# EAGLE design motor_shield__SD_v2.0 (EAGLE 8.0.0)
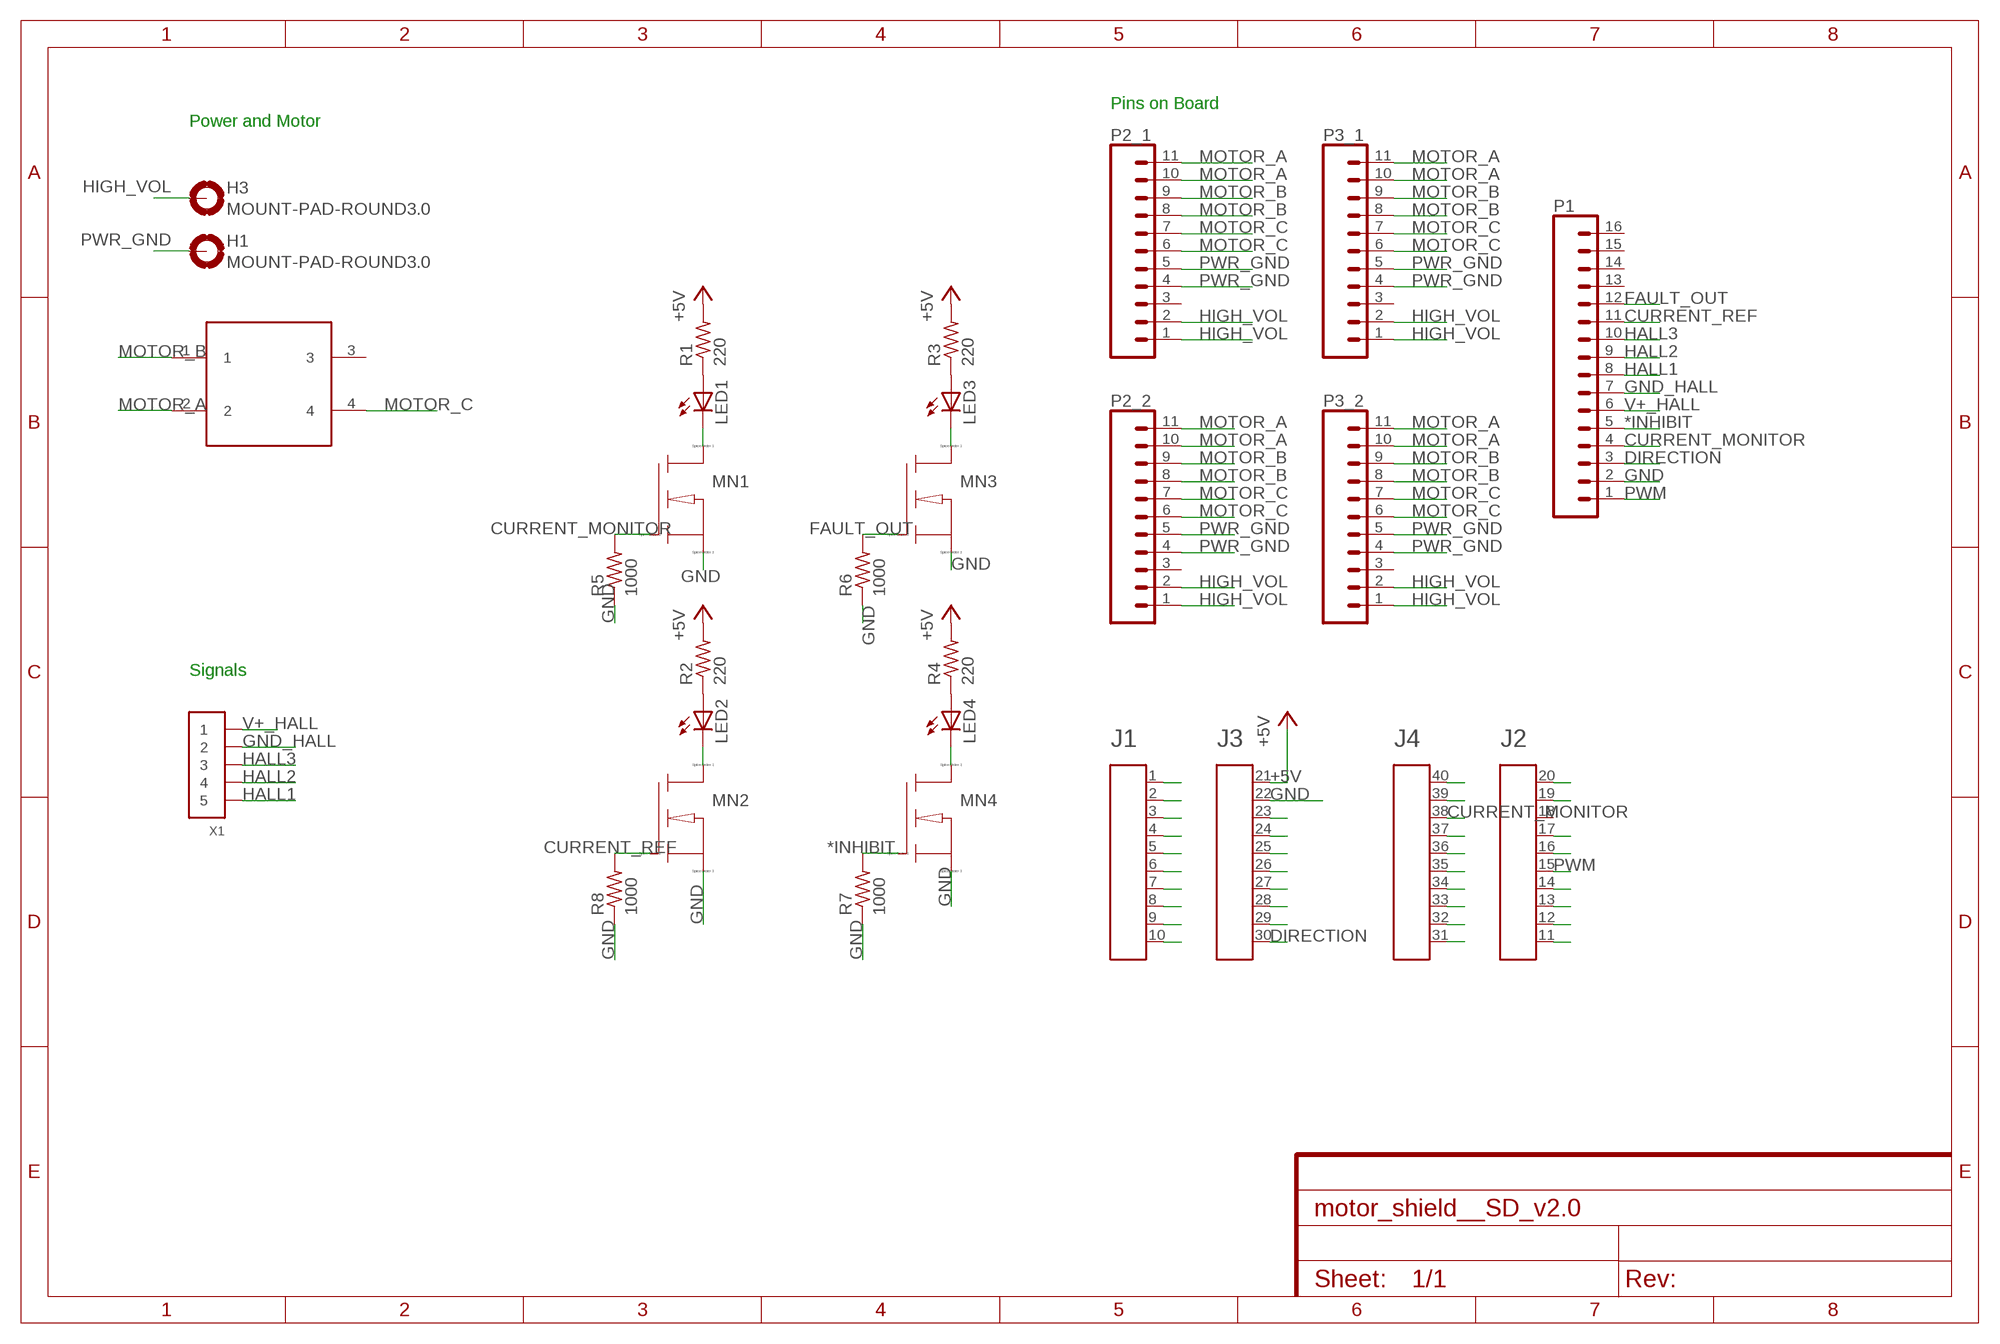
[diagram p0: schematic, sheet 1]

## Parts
A1  HEADER4X10-BOOSTERPACK  [4X10-BOOSTERPACK]
H1  MOUNT-PAD-ROUND3.0  [3,0-PAD]
H3  MOUNT-PAD-ROUND3.0  [3,0-PAD]
LED1  LEDCHIPLED_0805  [CHIPLED_0805]
LED2  LEDCHIPLED_0805  [CHIPLED_0805]
LED3  LEDCHIPLED_0805  [CHIPLED_0805]
LED4  LEDCHIPLED_0805  [CHIPLED_0805]
MN1  NMOS  [SOT23]
MN2  NMOS  [SOT23]
MN3  NMOS  [SOT23]
MN4  NMOS  [SOT23]
P1  CONN_16LOCK  [1X16_LOCK]
P2_1  CONN_11  [1X11]
P2_2  CONN_11  [1X11]
P3_1  CONN_11  [1X11]
P3_2  CONN_11  [1X11]
R1  220  R-US_R0603  [R0603]
R2  220  R-US_R0603  [R0603]
R3  220  R-US_R0603  [R0603]
R4  220  R-US_R0603  [R0603]
R5  1000  R-US_R0603  [R0603]
R6  1000  R-US_R0603  [R0603]
R7  1000  R-US_R0603  [R0603]
R8  1000  R-US_R0603  [R0603]
U$2  MOLEX4CON  [MOLEX4CON]
X1  CONN_5-1-53261  [PB-53261-05]

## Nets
*INHIBIT: MN4.1(G) P1.5 R7.2
+5V: A1.21 R1.2 R2.2 R3.2 R4.2
CURRENT_MONITOR: A1.38 MN1.1(G) P1.4 R5.2
CURRENT_REF: MN2.1(G) P1.11 R8.2
DIRECTION: A1.30 P1.3
FAULT_OUT: MN3.1(G) P1.12 R6.2
GND: A1.22 MN1.2(S) MN2.2(S) MN3.2(S) MN4.2(S) P1.2 R5.1 R6.1 R7.1 R8.1
GND_HALL: P1.7 X1.2
HALL1: P1.8 X1.5
HALL2: P1.9 X1.4
HALL3: P1.10 X1.3
HIGH_VOL: H3.B3,0(MOUNT) P2_1.1 P2_1.2 P2_2.1 P2_2.2 P3_1.1 P3_1.2 P3_2.1 P3_2.2
MOTOR_A: P2_1.10 P2_1.11 P2_2.10 P2_2.11 P3_1.10 P3_1.11 P3_2.10 P3_2.11 U$2.2
MOTOR_B: P2_1.8 P2_1.9 P2_2.8 P2_2.9 P3_1.8 P3_1.9 P3_2.8 P3_2.9 U$2.1
MOTOR_C: P2_1.6 P2_1.7 P2_2.6 P2_2.7 P3_1.6 P3_1.7 P3_2.6 P3_2.7 U$2.4
N$1: LED1.A R1.1
N$2: LED2.A R2.1
N$10: LED3.A R3.1
N$11: LED4.A R4.1
N$15: LED1.C MN1.3(D)
N$16: LED2.C MN2.3(D)
N$30: LED3.C MN3.3(D)
N$41: LED4.C MN4.3(D)
N$46: A1.1
N$47: A1.2
N$48: A1.3
N$49: A1.4
N$50: A1.5
N$51: A1.6
N$52: A1.7
N$53: A1.8
N$54: A1.9
N$55: A1.10
N$58: A1.23
N$59: A1.24
N$60: A1.25
N$61: A1.26
N$62: A1.27
N$63: A1.28
N$64: A1.29
N$66: A1.40
N$67: A1.39
N$69: A1.37
N$70: A1.36
N$71: A1.35
N$72: A1.34
N$73: A1.33
N$74: A1.32
N$75: A1.31
N$76: A1.20
N$77: A1.19
N$79: A1.17
N$80: A1.16
N$82: A1.14
N$83: A1.13
N$84: A1.12
N$85: A1.11
PWM: A1.15 P1.1
PWR_GND: H1.B3,0(MOUNT) P2_1.4 P2_1.5 P2_2.4 P2_2.5 P3_1.4 P3_1.5 P3_2.4 P3_2.5
V+_HALL: P1.6 X1.1
Unconnected: A1.18 P1.13 P1.14 P1.15 P1.16 P2_1.3 P2_2.3 P3_1.3 P3_2.3 U$2.3

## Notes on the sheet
- Pins on Board
- Power and Motor
- Signals

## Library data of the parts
A1 = EAGLE_BoosterPack_Library:HEADER4X10-BOOSTERPACK
H1 H3 = holes:MOUNT-PAD-ROUND: MOUNTING PAD, round
LED1-LED4 = adafruit:LED: LED
MN1-MN4 = sym:NMOS: N-Channel MOSFET transistor
P1 = SparkFun-Connectors:CONN_16: Multi connection point. Often used as Generic Header-pin footprint for 0.1 inch spaced/style header connections On any of the 0.1 inch spaced packages, you can populate with these: Break Away Headers - Straight (PRT-00116) Break Away Male Headers - Right Angle (PRT-00553) Female Headers (PRT-00115)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
P2_1 P2_2 P3_1 P3_2 = SparkFun-Connectors:CONN_11: Multi connection point. Often used as Generic Header-pin footprint for 0.1 inch spaced/style header connections On any of the 0.1 inch spaced packages, you can populate with these: Break Away Headers - Straight (PRT-00116) Break Away Male Headers - Right Angle (PRT-00553) Female Headers (PRT-00115)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
R1-R8 = adafruit:R-US_: RESISTOR, American symbol
U$2 = TREC1:MOLEX4CON
X1 = pel_molex:CONN_5-1

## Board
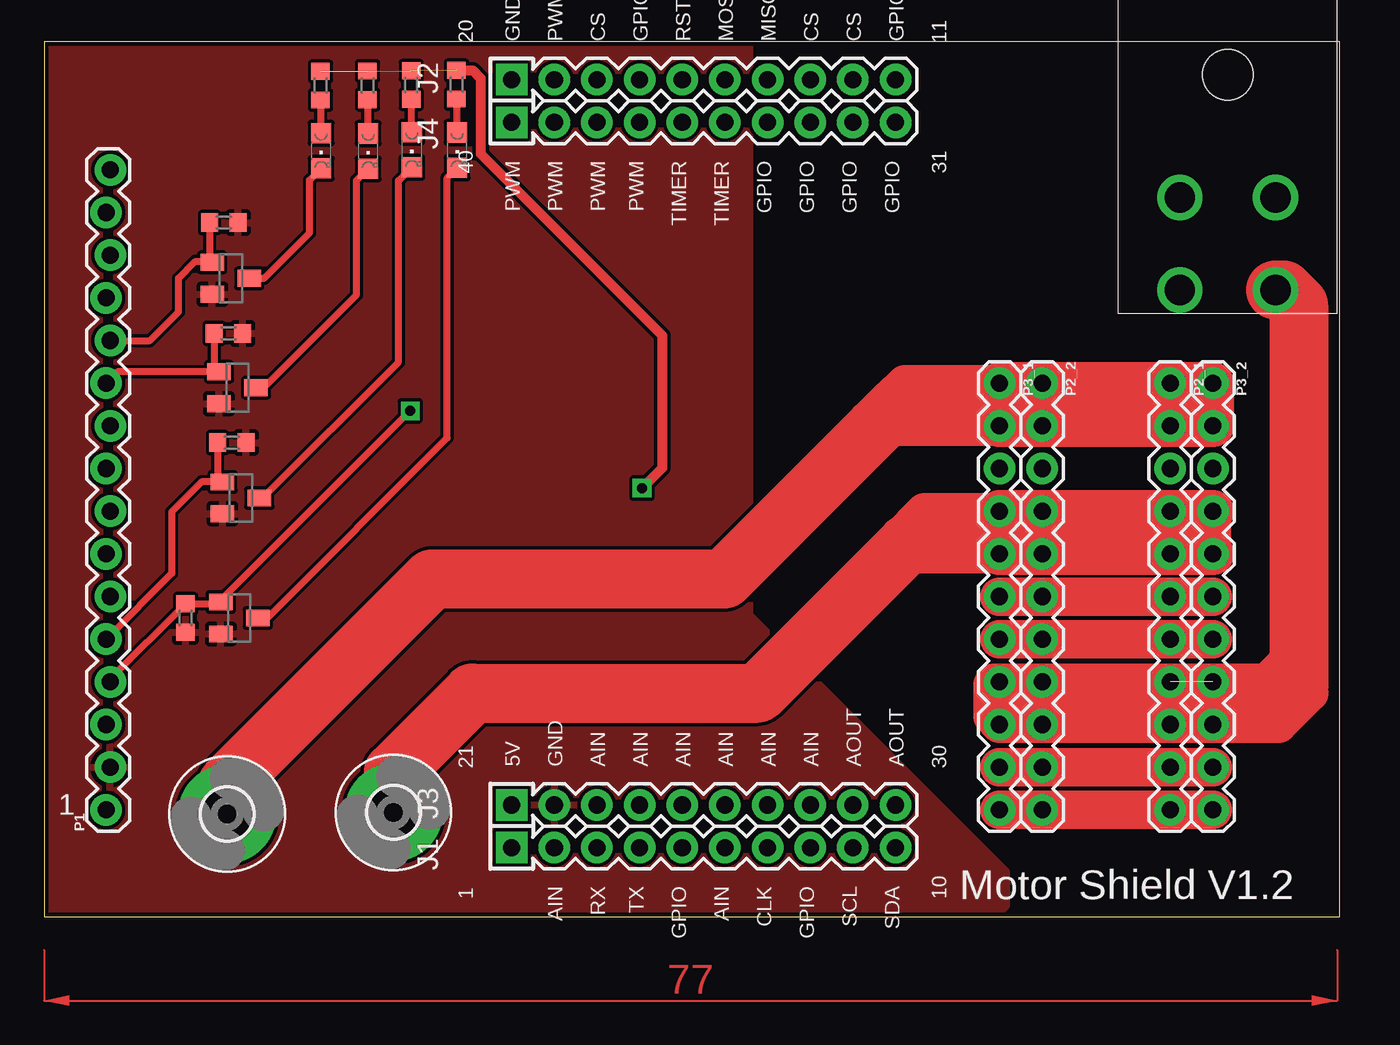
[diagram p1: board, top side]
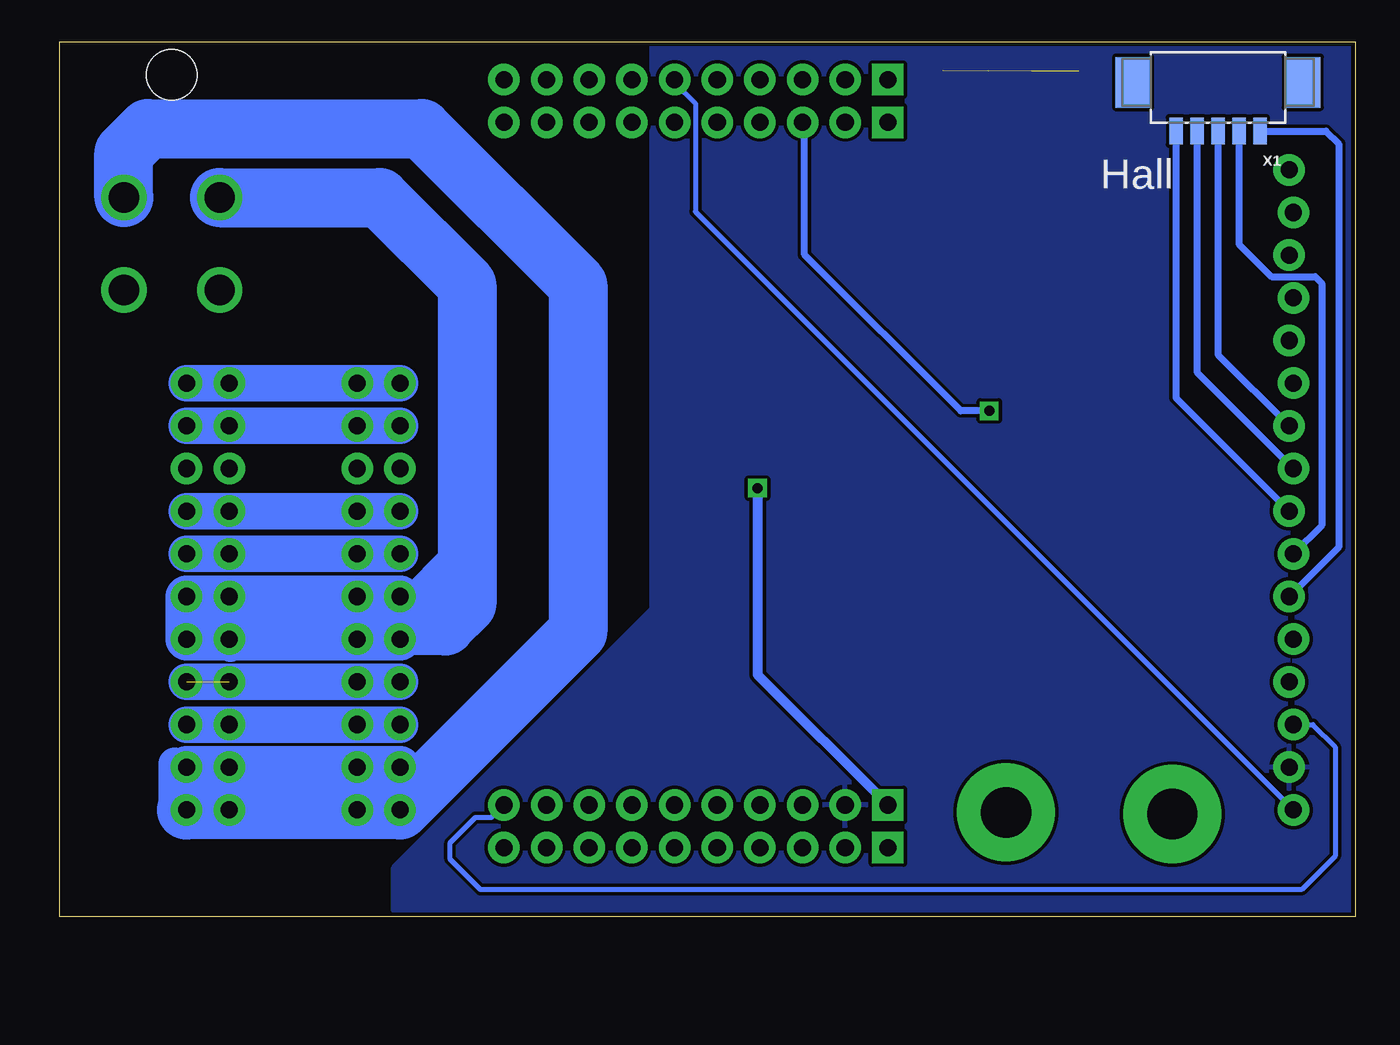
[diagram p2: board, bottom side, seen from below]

Size 77.14 x 52.06 mm. Coordinates in mm from the lower left corner, seen from the top.
Outline: 0,0 77.14,0 77.14,52.06 0,52.06 0,0
Copper layers (1*16): Top 0.035mm / dielectric 1.5mm / Bottom 0.035mm
Design rules "SparkFun": minimum track width 8mil, minimum drill 20mil, track to track 8mil, track to pad 8mil, pad to pad 8mil, via to via 8mil, smd to smd 8mil, copper to edge 10mil, drill to drill 8mil, minimum pad ring 12mil, minimum via ring 10mil, stop-mask expansion 4mil, vias tented up to drill 25mil, thermal gap 10mil

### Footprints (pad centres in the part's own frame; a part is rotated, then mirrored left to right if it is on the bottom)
4X10-BOOSTERPACK = drill 1.016 pad 1.88 square: 1 0,10.16; 20 45.72,10.16; 21 2.54,10.16; 40 43.18,10.16 | drill 1.016 pad 1.88: 2 0,7.62; 3 0,5.08; 4 0,2.54; 5 0,0; 6 0,-2.54; 7 0,-5.08; 8 0,-7.62; 9 0,-10.16; 10 0,-12.7; 11 45.72,-12.7; 12 45.72,-10.16; 13 45.72,-7.62; 14 45.72,-5.08; 15 45.72,-2.54; 16 45.72,0; 17 45.72,2.54; 18 45.72,5.08; 19 45.72,7.62; 22 2.54,7.62; 23 2.54,5.08; 24 2.54,2.54; 25 2.54,0; 26 2.54,-2.54; 27 2.54,-5.08; 28 2.54,-7.62; 29 2.54,-10.16; 30 2.54,-12.7; 31 43.18,-12.7; 32 43.18,-10.16; 33 43.18,-7.62; 34 43.18,-5.08; 35 43.18,-2.54; 36 43.18,0; 37 43.18,2.54; 38 43.18,5.08; 39 43.18,7.62
3,0-PAD = drill 3 pad 5.842: B3,0 0,0
CHIPLED_0805 = smd 1.2 x 1.2: A 0,-1.05; C 0,1.05
SOT23 = smd 1 x 1.4: 1 -0.95,-1.1; 2 0.95,-1.1; 3 0,1.1
1X16_LOCK = drill 1.016 pad 1.88: 1 0,0.127; 2 2.54,-0.127; 3 5.08,0.127; 4 7.62,-0.127; 5 10.16,0.127; 6 12.7,-0.127; 7 15.24,0.127; 8 17.78,-0.127; 9 20.32,0.127; 10 22.86,-0.127; 11 25.4,0.127; 12 27.94,-0.127; 13 30.48,0.127; 14 33.02,-0.127; 15 35.56,0.127; 16 38.1,-0.127
1X11 = drill 1.016 pad 1.88: 1 0,0; 2 2.54,0; 3 5.08,0; 4 7.62,0; 5 10.16,0; 6 12.7,0; 7 15.24,0; 8 17.78,0; 9 20.32,0; 10 22.86,0; 11 25.4,0
R0603 = smd 1 x 1.1: 1 -0.85,0; 2 0.85,0
MOLEX4CON = drill 1.8: 1 3.67,21.4; 2 3.67,15.9; 3 9.37,21.4; 4 9.37,15.9 | hole 3: 6.52,8.6
PB-53261-05 = smd 0.8 x 1.6: 1 -2.5,1.1; 2 -1.25,1.1; 3 0,1.1; 4 1.25,1.1; 5 2.5,1.1 | smd 2.1 x 3: MNT1 -5.05,-1.8; MNT2 5.05,-1.8

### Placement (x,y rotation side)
A1  38,4.1 90 top
H1  20.8,6.2 0 top
H3  10.9,6.1 0 top
LED1  24.59,45.63 180 top
LED2  19.29,45.57 180 top
LED3  16.49,45.59 180 top
LED4  21.89,45.65 180 top
MN1  11.62,17.77 270 top
MN2  11.52,31.48 270 top
MN3  11.12,37.99 270 top
MN4  11.72,24.92 270 top
P1  3.81,6.35 90 top
P2_1  67.06,31.75 270 top
P2_2  59.44,31.75 270 top
P3_1  56.9,31.75 270 top
P3_2  69.6,31.75 270 top
R1  24.56,49.52 90 top
R2  19.26,49.48 90 top
R3  16.46,49.46 90 top
R4  21.86,49.5 90 top
R5  8.41,17.77 90 top
R6  10.71,41.31 180 top
R7  11.18,28.21 180 top
R8  10.98,34.71 180 top
U$2  77,58.7 180 top
X1  8.18,47.86 180 bottom

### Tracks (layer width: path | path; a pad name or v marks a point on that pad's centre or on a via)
*INHIBIT
  Top 0.406: R7.2 10.33,26.16 MN4.1 9.37,25.87 7.6,24.1 7.6,20.43 P1.5
+5V  (via drill 0.6)  (3 unrouted)
  Top 0.61: R1.2 25.53,50.37 26,49.9 26,45.4 36.8,34.6 36.8,26.7 v35.6,25.5
  Bottom 0.61: v35.6,25.5 35.6,14.4 A1.21
CURRENT_MONITOR  (via drill 0.6)
  Top 0.406: P1.4 3.94,14.14 R5.2 10.42,18.62 MN1.1 10.52,18.82 v21.8,30.1
  Bottom 0.406: v21.8,30.1 23.5,30.1 32.8,39.4 32.8,47.16 A1.38
CURRENT_REF
  Top 0.406: R8.2 10.13,32.72 MN2.1 4.36,32.43 P1.11
DIRECTION
  Bottom 0.305: P1.3 2.53,11.43 1.2,10.1 1.2,3.6 3.2,1.6 52.1,1.6 53.9,3.4 53.9,4.4 52.4,5.9 51.44,5.9 A1.30
FAULT_OUT
  Top 0.406: R6.2 9.86,39.1 MN3.1 9.96,39 9,39 8,38 8,36 6.29,34.29 P1.12
GND
  pour Bottom: 0.1,52 41.9,52 41.9,27.7 41.9,18.3 51.7,8.5 57.3,2.9 57.3,0.4 57,0.1 0.1,0.1
  pour Top: 0.1,52 42,52 42,18 57.3,2.7 57.3,0.6 56.8,0.1 0.1,0.1
GND_HALL
  Bottom 0.406: X1.2 6.93,40.03 5,38.1 2.4,38.1 2,37.7 2,23.27 P1.7
HALL1
  Bottom 0.406: X1.5 10.68,30.87 P1.8
HALL2
  Bottom 0.406: X1.4 9.43,32.41 P1.9
HALL3
  Bottom 0.406: X1.3 8.18,33.45 P1.10
HIGH_VOL
  Top 2.184: P3_1.1 51.25,31.75 50.4,30.9 | 49.5,29.1 59.33,29.1 P2_2.2
  Top 2.54: P2_1.1 P3_1.1 P3_1.2 P2_2.2 | P2_2.2 P3_2.2 P3_2.1 P2_1.1 | P2_2.1 P2_2.2 | P2_1.2 P2_1.1
  Top 3.51: H3.B3,0 10.9,7.9 23.1,20.1 40.5,20.1 49.5,29.1 50.8,30.4 57.3,30.4 57.8,30.9 63.7,30.9 64.2,30.4 64.7,30.4 64.8,30.5 69,30.5
  Bottom 2.184: P3_2.1 P3_1.1 | P3_2.2 P3_1.2
MOTOR_A
  Top 2.3: P3_1.10 P3_2.10 | P3_1.11 P3_2.11
  Bottom 1.93: P3_2.11 69.6,8.4 70.3,9.1 70.3,6.1 70.2,6
  Bottom 2.3: 59.44,6.06 P2_2.10 P2_2.11 | P2_1.11 P3_2.10 P2_1.10
  Bottom 2.54: P3_1.11 P2_1.11 P3_2.11 | P3_1.10 P2_2.10 P3_2.10
  Bottom 3.51: P3_2.11 P3_1.11 46.3,16.95 46.3,37.6 55.6,46.9 71.9,46.9 73.33,45.47 U$2.2
MOTOR_B  (1 unrouted)
  Top 1.676: P2_2.8 58.44,13.97 56.4,11.93 | P3_1.8 P2_2.9 | P2_1.9 P3_2.9
  Top 2.184: 73.8,15 72.77,13.97 P3_2.8 P3_1.8 56.57,13.97 56.4,13.8 56.4,11.93 | 56.4,11.93 P3_1.9 P2_2.9 P3_2.9 73.53,11.43 75.4,13.3 | 56.4,11.93 69.13,11.93 69.9,12.7
  Top 3.51: U$2.1 73.8,37.3 74.7,36.4 74.7,13.6 73.8,12.7 69.9,12.7 57.3,12.7
  Bottom 2.184: P3_1.8 P3_2.8 | P3_1.9 P3_2.9
MOTOR_C
  Top 2.3: P3_1.6 P3_2.6 | P3_1.7 P3_2.7
  Bottom 1.676: P2_1.7 P3_2.7 | P3_2.6 69.6,18.6 67,16 67,16.1 68.1,17.2
  Bottom 1.93: 53.8,20 54.75,19.05 P3_1.6 55.85,19.05 53.9,21
  Bottom 2.54: 66.5,16.51 P3_2.7 P3_2.6 P2_1.6 | P2_2.7 66.5,16.51 | P3_1.7 P2_2.7 | P2_1.6 P3_1.6 P2_2.7 | P2_1.6 67.06,17.07 66.5,16.51 | P2_2.6 P2_2.7 | P2_1.6 P2_1.7
  Bottom 3.51: U$2.4 58.1,42.8 52.9,37.6 52.9,18.6 54.2,17.3 60.9,17.3 61,17.2 68.1,17.2 68.7,17.8
N$1
  Top 0.406: R1.1 24.56,46.71 LED1.A
N$2
  Top 0.406: R2.1 19.26,46.65 LED2.A
N$10
  Top 0.406: R3.1 16.46,46.67 LED3.A
N$11
  Top 0.406: R4.1 21.86,46.73 LED4.A
N$15
  Top 0.406: LED1.C 24,43.98 24,28.5 13.27,17.77 MN1.3
N$16
  Top 0.406: MN2.3 13.08,31.48 18.6,37 18.6,43.82 LED2.C
N$30
  Top 0.406: MN3.3 13.09,37.99 15.8,40.7 15.8,43.84 LED3.C
N$41
  Top 0.406: MN4.3 13.02,24.92 21.1,33 21.1,43.8 LED4.C
PWM
  Bottom 0.305: A1.15 40.54,49.64 39.3,48.4 39.3,41.97 P1.1
PWR_GND
  Top 2.184: P3_1.4 52.43,24.13 50.8,22.5 | P3_2.4 P3_2.5
  Top 2.54: P2_2.5 P3_1.5 P3_1.4 P2_2.4 | P2_1.5 P2_2.5 | P3_2.5 P2_1.5 | P2_2.4 P3_2.4 68.08,22.62 P2_1.5 | P2_2.4 P2_2.5 | P2_1.4 P2_1.5
  Top 3.51: H1.B3,0 20.8,8.6 25.5,13.3 42.5,13.3 51.4,22.2 67.67,22.2 68.08,22.62
  Bottom 2.184: P3_1.4 P3_2.4 | P3_1.5 P3_2.5
V+_HALL
  Bottom 0.406: X1.1 1.76,46.76 1,46 1,21.99 P1.6
(copper drawn outside any net)
  shapes: Top area x2

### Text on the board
tPlace: 1 | Motor Shield V1.2
bPlace: Hall

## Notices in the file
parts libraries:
SparkFun-Connectors: Licensing: Creative Commons ShareAlike 4.0 International - https://creativecommons.org/licenses/by-sa/4.0
